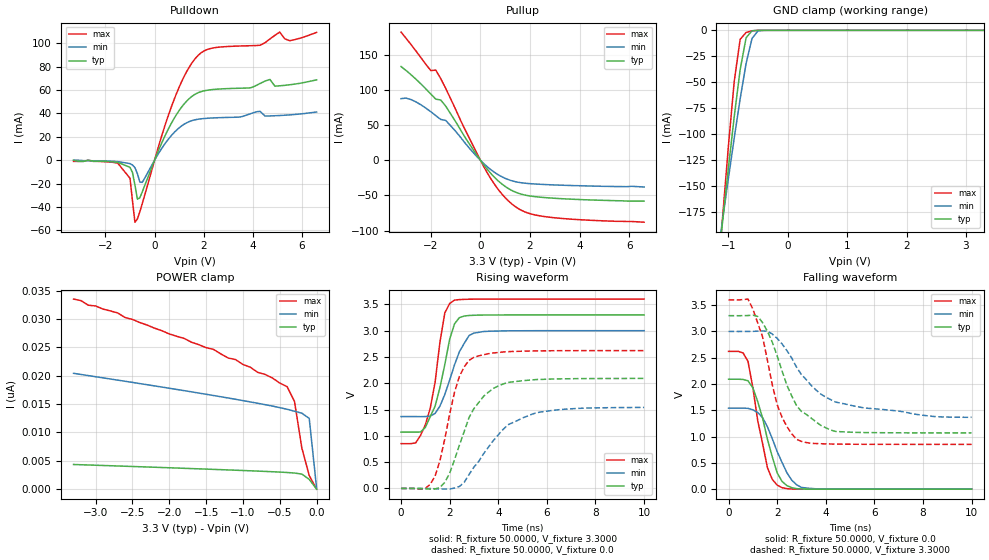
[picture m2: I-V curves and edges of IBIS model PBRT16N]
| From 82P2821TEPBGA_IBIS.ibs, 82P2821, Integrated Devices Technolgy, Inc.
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|   Model PBRT16N
[Model]		PBRT16N
Model_type	I/O
Polarity   Non-Inverting
Enable   Active-Low
Vinl = 		0.8000V
Vinh = 		2.0000V
C_comp   7.5800pF   7.4400pF   8.2500pF
[Temperature Range]	  25.0000   90.0000   -40.0000
[Voltage Range]   3.3000V   3.0000V   3.6000V
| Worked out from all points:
|   slope of the pulldown table from 0 to 0.495 V, typ, clamps not added: 20.7 ohm
|   slope of the pullup table from 0 to 0.495 V, typ, clamps not added: 22.9 ohm
|   GND clamp passes 1 mA (typ) near -0.61 V on its own axis
|   rising waveform, R_fixture 50.0000, V_fixture 3.3000: 20-80 % time 659ps typ, 777ps min, 574ps max; typ from 1.07 V to 3.3 V
|   rising waveform, R_fixture 50.0000, V_fixture 0.0: 20-80 % time 1.16ns typ, 1.64ns min, 782ps max; typ from 0 V to 2.09 V
|   falling waveform, R_fixture 50.0000, V_fixture 0.0: 20-80 % time 734ps typ, 860ps min, 616ps max; typ from 2.09 V to 0 V
|   falling waveform, R_fixture 50.0000, V_fixture 3.3000: 20-80 % time 1.19ns typ, 1.9ns min, 887ps max; typ from 3.3 V to 1.07 V
[Pulldown]
|Voltage	  I(typ)   I(min)   I(max)
-3.3V     0A         0A         -1mA
-1.5V     -1.8mA     -1.2mA     -2.5mA
-1V       -6.1mA     -2.9mA     -15.5mA
-800mV    -21.17mA   -6.34mA    -53.06mA
-700mV    -33.36mA   -11.46mA   -50.27mA
-500mV    -27.05mA   -18.95mA   -37.08mA
700mV     32.23mA    21.5mA     46.59mA
1.7V      57.04mA    34.83mA    88.11mA
4.7V      69.16mA    37.92mA    103.8mA
5.1V      63.72mA    38.28mA    109.7mA
5.5V      64.58mA    38.81mA    102.3mA
6.6V      68.79mA    41.26mA    109.4mA
[Pullup]
|Voltage	  I(typ)   I(min)   I(max)
-3.2V     133.1mA    87.54mA    182.1mA
-2.8V     121.6mA    86.26mA    164.5mA
-2V       94.07mA    68.92mA    127.3mA
-1.8V     86.81mA    63.42mA    128.1mA
-1.6V     85.57mA    57.97mA    116mA
-1.4V     76.95mA    56.62mA    102.2mA
200mV     -9.5mA     -6.821mA   -13.19mA
700mV     -28.75mA   -20.19mA   -40.59mA
1.3V      -43.51mA   -29.49mA   -63.03mA
1.9V      -50.17mA   -32.94mA   -74.78mA
2.6V      -53.03mA   -34.48mA   -80.08mA
6.6V      -58mA      -38mA      -88mA
[GND_clamp]
|Voltage	  I(typ)   I(min)   I(max)
-3.3V     -1.417A    -1.129A    -1.858A
-1.2V     -239.2mA   -225mA     -255.1mA
-1.1V     -185.7mA   -183.7mA   -182.6mA
-1V       -133.3mA   -143.1mA   -112.7mA
-900mV    -83.08mA   -103.5mA   -49.1mA
-800mV    -37.76mA   -65.73mA   -8.666mA
-700mV    -7.072mA   -31.8mA    -2.029mA
-600mV    -432.8uA   -7.706mA   -440.9uA
-500mV    -28.09uA   -557uA     -48.67uA
3.3V      910.5fA    13.74nA    -711.9pA
[POWER_clamp]
|Voltage	  I(typ)   I(min)   I(max)
-3.3V     4.35nA     20.42nA    33.51nA
-3.2V     4.305nA    20.22nA    33.24nA
-3.1V     4.264nA    20.02nA    32.43nA
-2.7V     4.087nA    19.22nA    31.06nA
-2.6V     4.042nA    19.02nA    30.25nA
-1.4V     3.488nA    16.51nA    24.64nA
-600mV    3.072nA    14.65nA    19.6nA
-400mV    2.938nA    14.08nA    18.07nA
-300mV    2.843nA    13.74nA    15.47nA
-200mV    2.66nA     13.39nA    7.238nA
-100mV    1.729nA    12.47nA    2.405nA
0V        930fA      202.7pA    668.8fA
[Ramp]
| variable   typ   min   max
dV/dt_r		1.2546/1.1429n   0.9240/1.6629n   1.5720/0.7767n
dV/dt_f		1.3380/1.2250n   0.9798/1.9517n   1.6489/0.8444n
R_load =	50.0000
[Rising Waveform]
R_fixture=	50.0000
V_fixture=	3.3000
V_fixture_min=	3.0000
V_fixture_max=	3.6000
|time   V(typ)   V(min)   V(max)
0s        1.07V      1.366V     851.7mV
600ps     1.07V      1.366V     865.3mV
1ns       1.161V     1.366V     1.209V
1.4ns     1.563V     1.426V     2.018V
1.6ns     1.917V     1.565V     2.784V
1.8ns     2.356V     1.786V     3.336V
2.2ns     3.129V     2.35V      3.58V
2.6ns     3.277V     2.759V     3.595V
3ns       3.292V     2.954V     3.598V
10ns      3.299V     2.999V     3.599V
[Rising Waveform]
R_fixture=	50.0000
V_fixture=	0.0
V_fixture_min=	0.0
V_fixture_max=	0.0
|time   V(typ)   V(min)   V(max)
0s        0V         0V         0V
1ns       -8.86mV    -366.6uV   646.7uV
1.4ns     -10.04mV   -5.586mV   235.6mV
1.8ns     114.5mV    -12.14mV   942.5mV
2.4ns     822.4mV    37.1mV     2.128V
3ns       1.519V     405.2mV    2.494V
3.6ns     1.831V     788.8mV    2.562V
4.4ns     2.014V     1.21V      2.6V
5.4ns     2.064V     1.414V     2.613V
10ns      2.091V     1.54V      2.62V
[Falling Waveform]
R_fixture=	50.0000
V_fixture=	0.0
V_fixture_min=	0.0
V_fixture_max=	0.0
|time   V(typ)   V(min)   V(max)
0s        2.091V     1.541V     2.621V
600ps     2.087V     1.542V     2.59V
800ps     2.062V     1.537V     2.431V
1.2ns     1.666V     1.458V     1.303V
1.6ns     949mV      1.186V     408.6mV
2ns       310.6mV    715.6mV    77.51mV
2.2ns     147.1mV    508.9mV    28.41mV
2.6ns     28.2mV     171mV      3.305mV
3ns       4.31mV     33.91mV    859.6uV
10ns      12.56uV    55.68uV    2.319uV
[Falling Waveform]
R_fixture=	50.0000
V_fixture=	3.3000
V_fixture_min=	3.0000
V_fixture_max=	3.6000
|time   V(typ)   V(min)   V(max)
0s        3.3V       3V         3.6V
800ps     3.303V     3V         3.616V
1ns       3.311V     3.002V     3.427V
1.4ns     3.168V     3.01V      2.898V
2ns       2.535V     2.868V     1.607V
2.4ns     1.978V     2.636V     1.191V
2.8ns     1.588V     2.318V     947.7mV
3.6ns     1.28V      1.887V     867.8mV
4.4ns     1.098V     1.657V     857.3mV
10ns      1.07V      1.367V     851.8mV
